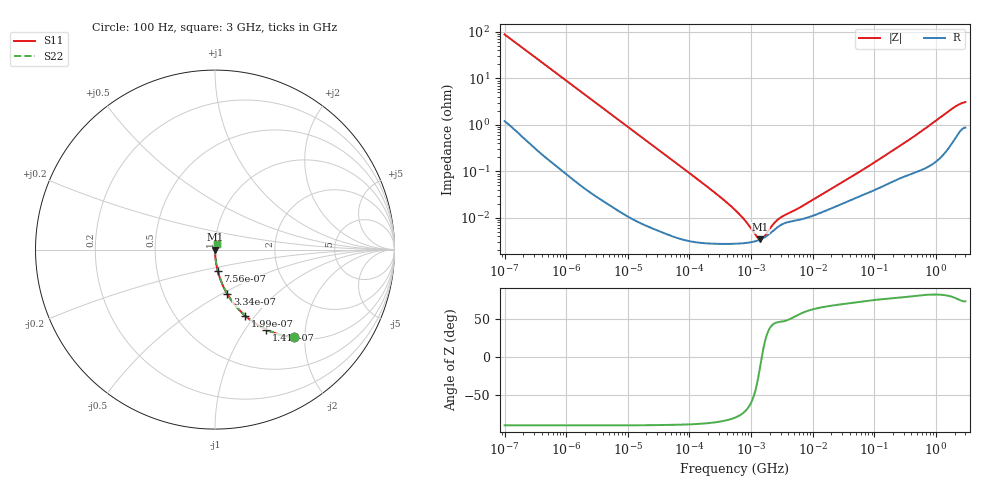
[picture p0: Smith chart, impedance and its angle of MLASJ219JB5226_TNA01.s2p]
! MLASJ219JB5226_TNA01  S-PARAMETER MODEL  ( Standard Model )
! Model Generated by TAIYO YUDEN Corporation (http://www.ty-top.com)
! Version 1.0
! TAIYO YUDEN Control No. 220601
! Copyright(c) 2009 TAIYO YUDEN CO.,LTD. All Rights Reserved.
! Product Description (link to TY-COMPAS)
! https://ds.yuden.co.jp/TYCOMPAS/or/detail?pn=MLASJ219JB5226MTNA01&u=M
! Products Name : Multilayer Ceramic Capacitors
! Characteristics :
!  Capacitance : 22 [uF] , Rated Voltage : 6.3 [V] , TCC : X5R
!  Case Size : 2.0 x 1.25 / 0.079 x 0.049 [mm/inch] , Thickness : 0.85 / 0.033 [mm/inch]
!  (Conditions: Temperature = 25 [degC] , DC Bias Voltage = 0 [V])
! External Node Assignments :
!  1  o---| |---o  2
! GND o---------o GND
! Frequency Range : 100Hz  -  3GHz  [ 401 STEP ]
# MHZ S RI R 50
! Freq[MHz].  S11 Real  S11 Imag  S21 Real  S21 Imag  S12 Real  S12 Imag  S22 Real  S22 Imag
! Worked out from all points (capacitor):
!   401 points, 100 Hz to 3 GHz, reference 50 ohm
!   read as one part in series: C = 18 uF near 109 Hz
!   lowest |Z| = 3.5 mohm at 1.412 MHz (marker M1)
!   series resonance near 1.488 MHz, so ESL is about 640 pH
!   S11 on the Smith chart (normalised r, x): 100 Hz: 1.02, -1.77; 141 Hz: 1.02, -1.26; 199 Hz: 1.01, -0.89; 334 Hz: 1.01, -0.54; 756 Hz: 1.00, -0.24; 3 GHz: 1.02, +0.06
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0.0001  0.4395 -0.4895  0.5605 0.4895  0.5605 0.4895  0.4395 -0.4895
0.000141  0.2859 -0.4454  0.7141 0.4454  0.7141 0.4454  0.2859 -0.4454
0.000199  0.1695 -0.3692  0.8305 0.3692  0.8305 0.3692  0.1695 -0.3692
0.000334  0.0691 -0.2484  0.9309 0.2484  0.9309 0.2484  0.0691 -0.2484
0.000756  0.015 -0.1168  0.985 0.1168  0.985 0.1168  0.015 -0.1168
0.001788  0.00301 -0.0503  0.997 0.0503  0.997 0.0503  0.00301 -0.0503
0.005476  0.000449 -0.0166  0.9996 0.0166  0.9996 0.0166  0.000449 -0.0166
0.031977  6.02e-05 -0.00287  0.9999 0.00287  0.9999 0.00287  6.02e-05 -0.00287
0.231582  2.81e-05 -0.00039  1 0.00039  1 0.00039  2.81e-05 -0.00039
0.547723  2.78e-05 -0.000146  1 0.000146  1 0.000146  2.78e-05 -0.000146
0.679242  2.82e-05 -0.000108  1 0.000108  1 0.000108  2.82e-05 -0.000108
0.772864  2.86e-05 -8.79e-05  1 8.79e-05  1 8.79e-05  2.86e-05 -8.79e-05
1.411895  3.44e-05 -6.56e-06  1 6.56e-06  1 6.56e-06  3.44e-05 -6.56e-06
2.93481  6.84e-05 7.24e-05  0.9999 -7.24e-05  0.9999 -7.24e-05  6.84e-05 7.24e-05
5.361412  8.8e-05 0.000123  0.9999 -0.000123  0.9999 -0.000123  8.8e-05 0.000123
9.794414  0.00011 0.000214  0.9999 -0.000214  0.9999 -0.000214  0.00011 0.000214
57.19833  0.00029 0.000936  0.9997 -0.000936  0.9997 -0.000936  0.00029 0.000936
175.1444  0.000565 0.00246  0.9994 -0.00246  0.9994 -0.00246  0.000565 0.00246
513.708  0.00104 0.00645  0.999 -0.00645  0.999 -0.00645  0.00104 0.00645
1950.712  0.00516 0.023  0.9948 -0.023  0.9948 -0.023  0.00516 0.023
2419.119  0.00776 0.0268  0.9922 -0.0268  0.9922 -0.0268  0.00776 0.0268
3000  0.00957 0.0293  0.9904 -0.0293  0.9904 -0.0293  0.00957 0.0293
